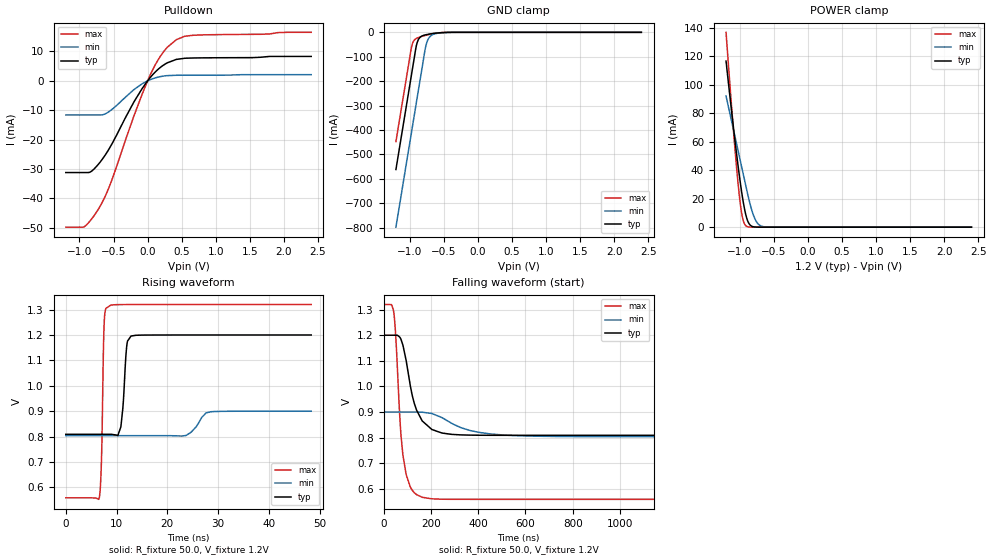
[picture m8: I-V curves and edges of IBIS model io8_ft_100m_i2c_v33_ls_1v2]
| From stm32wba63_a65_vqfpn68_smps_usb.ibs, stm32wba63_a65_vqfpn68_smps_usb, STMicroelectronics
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[Model]   io8_ft_100m_i2c_v33_ls_1v2
Model_type I/O_open_drain
Polarity   Non-Inverting
Enable   Active-Low
| CAP_THRESHOLD on pad IOFT is "UDTCAPC" :
| Rising=30.0% of vddiom   Falling=70.0% of vddiom
| C_comp min and max val. don't necessarily correlate with the min and max pvt
| but are the smallest and greatest pad capacitance found.
| var   typ   min   max
C_comp   2.87943pF  2.80398pF  2.98372pF
|C_comp_pulldown   2.87943pF  2.80398pF  2.98372pF
Vinl = 450.0mV
Vinh = 660.0mV
Vmeas = 600.0mV   | Reference voltage for timing measurements
Cref  = 50.0pF   | Timing specification test load capacitance value
Rref  = 1.0MOhm   | Timing specification test load resistance value
Vref  = 660.0mV   | Timing specification test load voltage
[Model Spec]
| TIME_THRESHOLD on pin ZII2CV11 is "CMOS" :
| Rising=50.0% of vdd   Falling=50.0% of vdd
Vinl 436.50000mV 331.50000mV 482.50000mV
Vinh 753.50000mV 549.50000mV 837.50000mV
| variable   typ   min   max
[Temperature Range] 25.0 140.0 -40.0
| variable   typ   min   max
[Voltage Range] 1.2V 900.0mV 1.32V
| variable   typ   min   max
[POWER Clamp Reference] 1.2V 900.0mV 1.32V
| variable   typ   min   max
[GND Clamp Reference] 0V 0V 0V
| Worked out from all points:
|   slope of the pulldown table from 0 to 0.18 V, typ, clamps not added: 40.6 ohm
|   GND clamp passes 1 mA (typ) near -0.51 V on its own axis
|   POWER clamp passes 1 mA (typ) near -0.83 V on its own axis
|   rising waveform, R_fixture 50.0, V_fixture 1.2V: 20-80 % time 743ps typ, 2.08ns min, 408ps max; typ from 0.809 V to 1.2 V
|   falling waveform, R_fixture 50.0, V_fixture 1.2V: 20-80 % time 60.2ns typ, 151ns min, 32.2ns max; typ from 1.2 V to 0.809 V
[POWER Clamp]
-1.2V     116.7mA    92.13mA    136.9mA
-1.09V    69.42mA    68.21mA    67.14mA
-1.02V    41.75mA    52.99mA    28.91mA
-990mV    30.98mA    46.47mA    16.09mA
-970mV    24.36mA    42.12mA    9.575mA
-940mV    15.59mA    35.6mA     3.485mA
-910mV    8.693mA    29.07mA    1.01mA
-860mV    2.259mA    18.59mA    104.6uA
-780mV    143.1uA    6.246mA    2.555uA
-720mV    16.22uA    1.846mA    157.1nA
-650mV    1.267uA    330.3uA    6.118nA
2.4V      0A         0A         0A
[GND Clamp]
-1.2V     -561.6mA   -797.4mA   -447.4mA
-980mV    -187.6mA   -423.4mA   -73.43mA
-960mV    -153.6mA   -389.4mA   -48.26mA
-900mV    -54.17mA   -287.4mA   -24.97mA
-870mV    -29.55mA   -236.4mA   -21.19mA
-830mV    -17.05mA   -168.4mA   -17.42mA
-760mV    -9.921mA   -54.55mA   -11.89mA
-730mV    -8.191mA   -29.78mA   -9.811mA
-690mV    -6.26mA    -14.49mA   -7.318mA
-600mV    -2.976mA   -4.315mA   -3.058mA
-380mV    -57.63uA   -251uA     -19.49uA
2.4V      872.8pA    204.8nA    349.4pA
| variable   typ   min   max
[Pullup Reference] 1.2V 900.0mV 1.32V
| variable   typ   min   max
[Pulldown Reference] 0V 0V 0V
[Pulldown]
-1.2V     -31.2mA    -11.62mA   -49.78mA
-930mV    -31.2mA    -11.62mA   -49.64mA
-830mV    -30.86mA   -11.62mA   -47.25mA
-710mV    -28.04mA   -11.62mA   -43.19mA
-550mV    -22.55mA   -10.2mA    -35.3mA
-200mV    -7.146mA   -2.964mA   -11.89mA
40mV      1.171mA    405.8uA    2.092mA
130mV     3.416mA    1.118mA    6.182mA
230mV     5.302mA    1.613mA    9.763mA
420mV     7.288mA    1.898mA    13.99mA
670mV     7.779mA    1.924mA    15.51mA
2.4V      8.312mA    2.101mA    16.51mA
[Ramp]
dV/dt_r 234.64839mV/730.90589ps 57.85686mV/2.00993ns 456.72359mV/405.98796ps
dV/dt_f 234.65961mV/57.80494ns 57.89301mV/147.8228ns 456.73576mV/31.47338ns
R_load = 50.0
| Removed startup time: 0s 0s 0s  .
| Removed end time: 48.35ns.
[Rising Waveform]
R_fixture   = 50.0
V_fixture   = 1.2V
V_fixture_min = 900.0mV
V_fixture_max = 1.32V
0s        808.9mV    803.5mV    558.8mV
6.6ns     808.9mV    803.5mV    559.4mV
7.05ns    808.9mV    803.5mV    723mV
7.5ns     808.9mV    803.5mV    1.214V
7.9ns     808.9mV    803.5mV    1.305V
10.85ns   838.4mV    803.5mV    1.32V
12ns      1.155V     803.5mV    1.32V
12.85ns   1.196V     803.5mV    1.32V
28.65ns   1.2V       897.8mV    1.32V
48.35ns   1.2V       899.9mV    1.32V
| Removed startup time: 0s 0s 0s  .
| Removed end time: 1.99825us.
[Falling Waveform]
R_fixture   = 50.0
V_fixture   = 1.2V
V_fixture_min = 900.0mV
V_fixture_max = 1.32V
0s        1.2V       900mV      1.32V
43.25ns   1.2V       900mV      1.286V
52.25ns   1.2V       900mV      1.179V
72.75ns   1.185V     900mV      816.9mV
95ns      1.102V     900mV      656.3mV
129.5ns   933.9mV    900mV      584.8mV
163.3ns   865mV      899.2mV    566.8mV
250.7ns   817.3mV    875.9mV    559.2mV
530.3ns   808.9mV    808.9mV    558.8mV
1.998us   808.9mV    803.5mV    558.8mV
